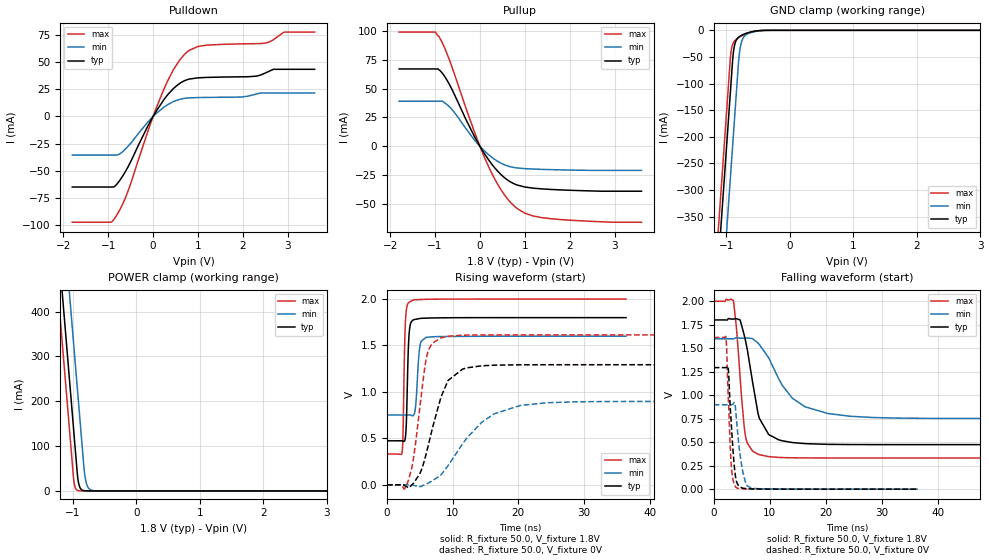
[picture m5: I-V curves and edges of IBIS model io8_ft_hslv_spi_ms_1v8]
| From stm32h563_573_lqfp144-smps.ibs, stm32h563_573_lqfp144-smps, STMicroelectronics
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[Model]   io8_ft_hslv_spi_ms_1v8
Model_type I/O
Polarity   Non-Inverting
Enable   Active-Low
| CAP_THRESHOLD on pad IOFT is "UDTCAPC" :
| Rising=20.0% of vddiom   Falling=80.0% of vddiom
| C_comp min and max val. don't necessarily correlate with the min and max pvt
| but are the smallest and greatest pad capacitance found.
| var   typ   min   max
C_comp   4.56172pF  4.45460pF  4.74994pF
|C_comp_pullup   2.85885pF  2.67925pF  2.77980pF
|C_comp_pulldown   1.70287pF  1.77535pF  1.97014pF
Vinl = 480.0mV
Vinh = 1.4V
Vmeas = 900.0mV   | Reference voltage for timing measurements
Cref  = 50.0pF   | Timing specification test load capacitance value
Rref  = 100.0MOhm   | Timing specification test load resistance value
Vref  = 900.0mV   | Timing specification test load voltage
[Model Spec]
| TIME_THRESHOLD on pin ZIV11 is "CMOS" :
| Rising=40.0% of vdd   Falling=60.0% of vdd
Vinl 703.80000mV 631.80000mV 784.80000mV
Vinh 1.06220V 937.20000mV 1.16620V
| variable   typ   min   max
[Temperature Range] 25.0 125.0 -40.0
| variable   typ   min   max
[Voltage Range] 1.8V 1.6V 2.0V
| variable   typ   min   max
[POWER Clamp Reference] 1.8V 1.6V 2.0V
| variable   typ   min   max
[GND Clamp Reference] 0V 0V 0V
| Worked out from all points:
|   slope of the pulldown table from 0 to 0.27 V, typ, clamps not added: 15.8 ohm
|   slope of the pullup table from 0 to 0.27 V, typ, clamps not added: 17.1 ohm
|   GND clamp passes 1 mA (typ) near -0.52 V on its own axis
|   POWER clamp passes 1 mA (typ) near -0.84 V on its own axis
|   rising waveform, R_fixture 50.0, V_fixture 1.8V: 20-80 % time 310ps typ, 455ps min, 283ps max; typ from 0.474 V to 1.8 V
|   falling waveform, R_fixture 50.0, V_fixture 1.8V: 20-80 % time 2.46ns typ, 5.75ns min, 1.32ns max; typ from 1.8 V to 0.474 V
|   rising waveform, R_fixture 50.0, V_fixture 0V: 20-80 % time 3.08ns typ, 6.35ns min, 1.7ns max; typ from 0 V to 1.29 V
|   falling waveform, R_fixture 50.0, V_fixture 0V: 20-80 % time 838ps typ, 1.11ns min, 637ps max; typ from 1.29 V to 0 V
[POWER Clamp]
-1.8V     1.518A     1.709A     1.407A
-1.23V    548.8mA    740.2mA    437.5mA
-1.16V    429.8mA    621.2mA    318.5mA
-1.05V    242.8mA    434.2mA    131.5mA
-980mV    123.8mA    315.2mA    17.95mA
-930mV    38.81mA    230.2mA    1.49mA
-910mV    17.82mA    196.2mA    550.8uA
-890mV    8.18mA     162.2mA    203.5uA
-810mV    363.5uA    33.6mA     3.797uA
-770mV    76.62uA    10.47mA    518.8nA
-710mV    7.417uA    1.822mA    26.38nA
3.6V      0A         0A         0A
[GND Clamp]
-1.8V     -1.581A    -1.742A    -1.516A
-1.24V    -628.8mA   -789.9mA   -564.1mA
-1.05V    -305.8mA   -466.9mA   -241.1mA
-940mV    -118.8mA   -279.9mA   -54.1mA
-930mV    -101.8mA   -262.9mA   -41.86mA
-900mV    -51.51mA   -211.9mA   -25.34mA
-880mV    -32.22mA   -177.9mA   -21mA
-810mV    -13.02mA   -59.5mA    -13.82mA
-770mV    -9.8mA     -24.99mA   -11mA
-680mV    -5.275mA   -7.288mA   -5.917mA
-400mV    -107uA     -349.1uA   -42.51uA
3.6V      5.392nA    968.2nA    261.3pA
| variable   typ   min   max
[Pullup Reference] 1.8V 1.6V 2.0V
| variable   typ   min   max
[Pulldown Reference] 0V 0V 0V
[Pullup]
-1.8V     66.99mA    38.98mA    98.93mA
-990mV    66.99mA    38.98mA    98.93mA
-920mV    66.55mA    38.98mA    95.61mA
-830mV    62.94mA    38.98mA    89.05mA
-650mV    51.43mA    33.05mA    71.74mA
-120mV    8.364mA    5.386mA    12.19mA
190mV     -11.56mA   -7.18mA    -17.34mA
510mV     -25.96mA   -15.42mA   -40.03mA
830mV     -33.6mA    -18.8mA    -53.95mA
1.18V     -36.29mA   -19.75mA   -60.37mA
1.56V     -37.38mA   -20.24mA   -62.7mA
3.6V      -38.97mA   -20.89mA   -65.81mA
[Pulldown]
-1.8V     -65.02mA   -35.56mA   -97.42mA
-940mV    -65.02mA   -35.56mA   -97.42mA
-850mV    -64.17mA   -35.56mA   -93.5mA
-570mV    -47.32mA   -28.01mA   -70.04mA
-120mV    -9.088mA   -5.279mA   -14.07mA
250mV     16.04mA    8.832mA    26.05mA
550mV     29.17mA    15.25mA    49.41mA
780mV     34.17mA    17.07mA    60.14mA
1.18V     35.97mA    17.56mA    65.65mA
2.49V     39.87mA    21.59mA    67.54mA
2.92V     43.47mA    21.59mA    77.77mA
3.6V      43.47mA    21.59mA    77.77mA
[Ramp]
dV/dt_r 775.81637mV/3.01026ns 538.93981mV/6.2163ns 968.32541mV/1.70242ns
dV/dt_f 795.78716mV/2.40346ns 508.97889mV/5.49061ns 1.00099V/1.32114ns
R_load = 50.0
| Removed startup time: 0s 0s 0s  .
| Removed end time: 36.4ns.
[Rising Waveform]
R_fixture   = 50.0
V_fixture   = 1.8V
V_fixture_min = 1.6V
V_fixture_max = 2.0V
0s        473.7mV    751.7mV    331.7mV
2.3ns     473.9mV    751.7mV    348.3mV
2.45ns    471.3mV    751.7mV    563.4mV
2.65ns    468.9mV    751.8mV    1.367V
2.8ns     507.1mV    751.8mV    1.74V
3.4ns     1.649V     752.1mV    1.966V
4.2ns     1.78V      771.4mV    1.992V
5ns       1.791V     1.483V     1.995V
5.95ns    1.795V     1.588V     1.997V
36.4ns    1.8V       1.6V       2V
| Removed startup time: 0s 0s 0s  .
| Removed end time: 199.4ns.
[Falling Waveform]
R_fixture   = 50.0
V_fixture   = 1.8V
V_fixture_min = 1.6V
V_fixture_max = 2.0V
0s        1.8V       1.6V       2V
3.5ns     1.81V      1.599V     2.003V
4.05ns    1.813V     1.611V     1.709V
4.7ns     1.797V     1.606V     1.19V
5.75ns    1.554V     1.607V     537.9mV
7.9ns     804.1mV    1.554V     371.9mV
9.8ns     581mV      1.397V     346.2mV
14.05ns   495.6mV    965.8mV    333.6mV
24.4ns    474.6mV    775mV      331.7mV
199.4ns   473.7mV    751.7mV    331.7mV
| Removed startup time: 0s 0s 0s  .
| Removed end time: 199.3ns.
[Rising Waveform]
R_fixture   = 50.0
V_fixture   = 0V
V_fixture_min = 0V
V_fixture_max = 0V
0s        134.7nV    547.1nV    93.86nV
3.1ns     -23.92mV   -36.75uV   15.92mV
4ns       14.43mV    -3.529mV   269.4mV
6.1ns     370.4mV    12.54mV    1.397V
7ns       632mV      48.45mV    1.528V
9.3ns     1.123V     205.7mV    1.6V
11.5ns    1.246V     440.1mV    1.611V
16.3ns    1.288V     763.5mV    1.614V
24.4ns    1.293V     883.7mV    1.614V
199.3ns   1.293V     898.2mV    1.614V
| Removed startup time: 0s 0s 0s  .
| Removed end time: 36.4ns.
[Falling Waveform]
R_fixture   = 50.0
V_fixture   = 0V
V_fixture_min = 0V
V_fixture_max = 0V
0s        1.293V     898.3mV    1.614V
2.15ns    1.293V     898.3mV    1.62V
2.3ns     1.296V     898.3mV    1.494V
2.6ns     1.274V     898.3mV    963.7mV
3.1ns     725.5mV    898.2mV    271.4mV
3.75ns    193.6mV    913.9mV    39.96mV
4.05ns    84.9mV     741.3mV    15.5mV
5.2ns     10.54mV    178.3mV    3.382mV
6.7ns     3.191mV    11.78mV    1.532mV
36.4ns    38.31nV    7.504uV    -120.9nV
